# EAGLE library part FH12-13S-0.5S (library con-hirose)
0.5mm Pitch Connectors For FPC/FFC Source: Data sheet
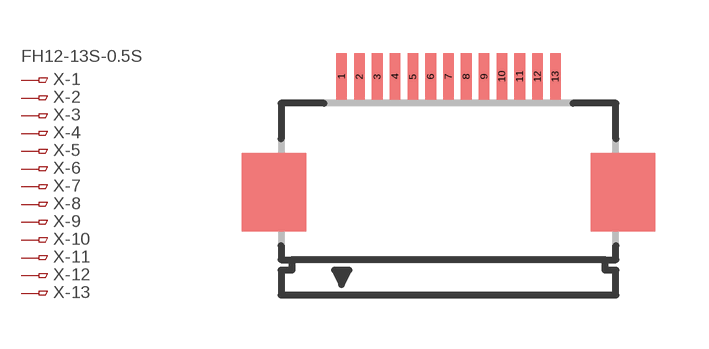
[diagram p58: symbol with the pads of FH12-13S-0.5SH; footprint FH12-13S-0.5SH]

Designator prefix X; gates -1=PINV -2=PIN -3=PIN -4=PIN -5=PIN -6=PIN -7=PIN -8=PIN -9=PIN -10=PIN -11=PIN -12=PIN -13=PIN

## FH12-13S-0.5SH (OC_FARNELL: 1324543; OC_NEWARK: unknown)  [FH12-13S-0.5SH]
1  -1:1  pas
2  -2:1  pas
3  -3:1  pas
4  -4:1  pas
5  -5:1  pas
6  -6:1  pas
7  -7:1  pas
8  -8:1  pas
9  -9:1  pas
10  -10:1  pas
11  -11:1  pas
12  -12:1  pas
13  -13:1  pas

## Footprint FH12-13S-0.5SH (pad centres in mm)
0.5mm Pitch Connectors For FPC/FFC Source: Data sheet
smd 0.3 x 1.3: 1 -3,3.25; 2 -2.5,3.25; 3 -2,3.25; 4 -1.5,3.25; 5 -1,3.25; 6 -0.5,3.25; 7 0,3.25; 8 0.5,3.25; 9 1,3.25; 10 1.5,3.25; 11 2,3.25; 12 2.5,3.25; 13 3,3.25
